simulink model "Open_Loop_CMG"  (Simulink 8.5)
settings: Solver=ode45  StartTime=0.0  StopTime=10000  FixedStep=Ts*5  RelTol=1e-3
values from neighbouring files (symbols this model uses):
  J = [0.119416e9, -0.476e7,   -0.1216e7;     -0.476e7,     0.40408e8, -0.30121e6;     -0.1216e7,   -0.30121e6,  0.110166e9]    [start.m]    (also in start1.m; start2.m; start3.m)
  omg = 20*wo    (= 0.022)    [start.m]    (also in start1.m; start2.m; start3.m)
  wo = 0.0011    [start.m]    (also in start1.m; start2.m; start3.m)
  zeb = 0.95    [start.m]    (also in start1.m; start2.m; start3.m)
undefined symbols (not defined in the file or in its folder): Af, Bf, Cf, Df

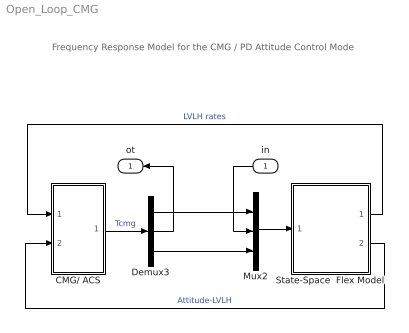
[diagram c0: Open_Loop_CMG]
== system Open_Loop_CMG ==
  note: Frequency Response Model for the CMG / PD Attitude Control Mode
  in : Inport
  CMG/ ACS : Subsystem
  Demux3 : Demux  Outputs=3
  Mux2 : Mux  Inputs=3
  State-Space  Flex Model : Subsystem
  ot : Outport
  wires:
  State-Space  Flex Model/1(w-lv) -> CMG/ ACS/1(wl)  "LVLH rates"
  State-Space  Flex Model/2(att-lv) -> CMG/ ACS/2(ater)  "Attitude-LVLH"
  CMG/ ACS/1(Tq) -> Demux3/1  "Tcmg"
  Mux2/1 -> State-Space  Flex Model/1(Tcmg)
  Demux3/3 -> Mux2/3
  Demux3/1 -> Mux2/1
  Demux3/2 -> ot/1
  in/1 -> Mux2/2

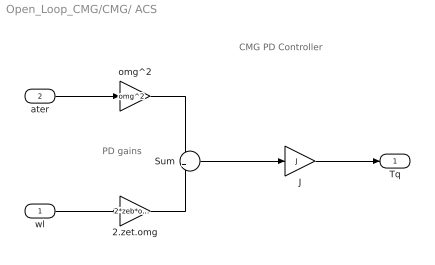
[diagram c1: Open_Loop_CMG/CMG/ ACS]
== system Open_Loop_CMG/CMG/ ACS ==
  note: CMG PD Controller
  note: PD gains
  wl : Inport
  ater : Inport  Port=2  PortDimensions=3
  2.zet.omg : Gain  Gain=2*zeb*omg
  J : Gain  Gain=J  Multiplication=Matrix(K*u)
  Sum : Sum
  omg^2 : Gain  Gain=omg^2
  Tq : Outport
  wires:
  wl/1 -> 2.zet.omg/1
  Sum/1 -> J/1
  2.zet.omg/1 -> Sum/2
  ater/1 -> omg^2/1
  omg^2/1 -> Sum/1
  J/1 -> Tq/1

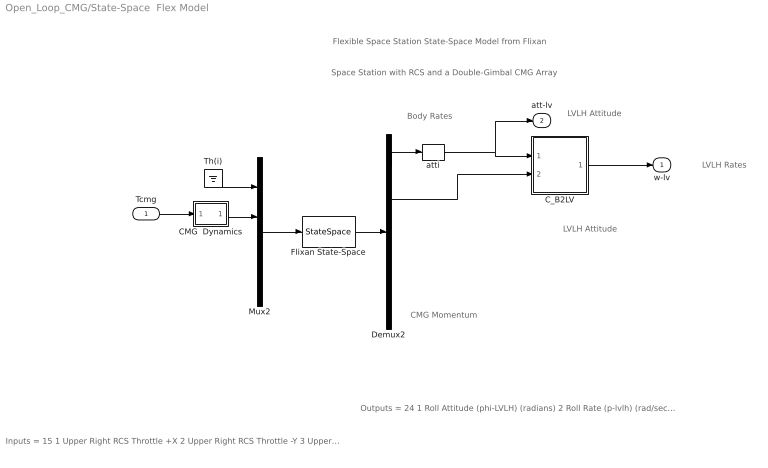
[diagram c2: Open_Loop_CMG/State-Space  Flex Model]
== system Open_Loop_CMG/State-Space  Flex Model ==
  note: Flexible Space Station State-Space Model from Flixan
  note: Space Station with RCS and a Double-Gimbal CMG Array
  note: Body Rates
  note: LVLH Attitude
  note: LVLH Rates
  note: Outputs = 24 1 Roll Attitude (phi-LVLH) (radians) 2 Roll Rate (p-lvlh) (rad/sec) 3 Pitch Attitude (thet-LVLH) (radians) 4 Pitch Rate (q-lvlh) (rad/sec) 5 Yaw Attitude (psi-LVLH) (radians) 6 Yaw Rate (r-lvlh) (rad/sec) 7 Angle of attack, alfa, (radians) 8 Angle of sideslip, beta, (radian) 9 Change in Altitude, delta-h, (feet) 10 Forward Acceleration (V-dot) (ft/sec) 11 Cross Range Velocity (Vcr) (ft/sec) 12 Rate-Gyro # 1, Roll Rate (Body) (rad/sec) 13 Rate-Gyro # 2, Pitch Rate (Body) (rad/sec) 14 Rate-Gyro # 3, Yaw Rate (Body) (rad/sec) 15 Gyro # 4, Roll Attitude (Body) (radians) 16 Gyro # 5, Pitch Attitude (Body) (radians) 17 Gyro # 6, Yaw Attitude (Body) (radians) 18 Accelerom # 1, (along X), (ft/sec^2) Translat. Accelerat. 19 Accelerom # 2, (along Z), (ft/sec^2) Translat. Accelerat. 20 Accelerom # 3, (along X), (ft/sec^2) Translat. Accelerat. 21 Accelerom # 4, (along Z), (ft/sec^2) Translat. Accelerat. 22 Double Gimbal CMG Momentum Change in X-axis (ft-lb-sec) 23 Double Gimbal CMG Momentum Change in Y-axis (ft-lb-sec) 24 Double Gimbal CMG Momentum Change in Z-axis (ft-lb-sec)
  note: LVLH Attitude
  note: Inputs = 15 1 Upper Right RCS Throttle +X 2 Upper Right RCS Throttle -Y 3 Upper Left RCS Throttle +X 4 Upper Left RCS Throttle +Y 5 Lower Right RCS Throttle +X 6 Lower Right RCS Throttle -Y 7 Lower Left RCS Throttle +X 8 Lower Left RCS Throttle +Y 9 Double Gimbal CMG Torque in the X-axis (ft-lb) 10 Double Gimbal CMG Torque in the Y-axis (ft-lb) 11 Double Gimbal CMG Torque in the Z-axis (ft-lb) 12 External Torque Input 1 (ft-lb), direct: 13 External Torque Input 2 (ft-lb), direct: 14 External Torque Input 3 (ft-lb), direct: 15 Ext Torque Direct.=(0.197, -0.5964, -0.7782)
  note: CMG Momentum
  Tcmg : Inport  PortDimensions=3
  CMG  Dynamics : Subsystem
  C_B2LV : Subsystem
  Demux2 : Demux  Outputs=[11, 3, 3, 4, 3]
  Flixan State-Space : StateSpace  A=Af  B=Bf  C=Cf  D=Df  X0=0
  Mux2 : Mux  Inputs=[8, 3, 3, 1]
  Th(i) : Ground
  atti : Selector  InputPortWidth=11  Indices=[1 3 5]
  w-lv : Outport
  att-lv : Outport  Port=2
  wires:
  Mux2/1 -> Flixan State-Space/1
  Flixan State-Space/1 -> Demux2/1
  Tcmg/1 -> CMG  Dynamics/1(I)
  Th(i)/1 -> Mux2/1
  Demux2/1 -> atti/1
  CMG  Dynamics/1(O) -> Mux2/2
  atti/1 -> att-lv/1, C_B2LV/1(atti)
  Demux2/2 -> C_B2LV/2(wb)
  C_B2LV/1(wlv) -> w-lv/1

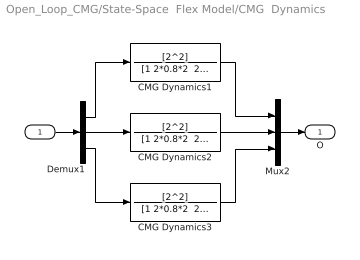
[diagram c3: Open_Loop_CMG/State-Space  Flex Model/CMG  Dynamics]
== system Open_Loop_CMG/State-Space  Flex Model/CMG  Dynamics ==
  I : Inport
  CMG Dynamics1 : TransferFcn  Numerator=[2^2]  Denominator="[1 2*0.8*2  2^2]"
  CMG Dynamics2 : TransferFcn  Numerator=[2^2]  Denominator="[1 2*0.8*2  2^2]"
  CMG Dynamics3 : TransferFcn  Numerator=[2^2]  Denominator="[1 2*0.8*2  2^2]"
  Demux1 : Demux  Outputs=3
  Mux2 : Mux  Inputs=3
  O : Outport
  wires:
  Mux2/1 -> O/1
  I/1 -> Demux1/1
  Demux1/3 -> CMG Dynamics3/1
  Demux1/1 -> CMG Dynamics1/1
  Demux1/2 -> CMG Dynamics2/1
  CMG Dynamics1/1 -> Mux2/1
  CMG Dynamics3/1 -> Mux2/3
  CMG Dynamics2/1 -> Mux2/2

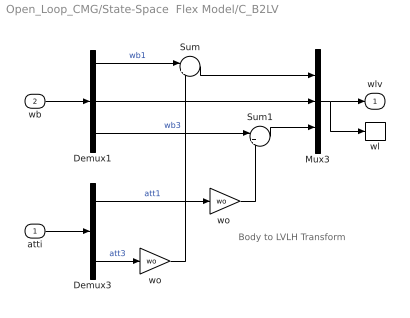
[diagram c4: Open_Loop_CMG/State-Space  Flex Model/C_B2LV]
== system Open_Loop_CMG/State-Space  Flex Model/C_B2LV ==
  note: Body to LVLH Transform
  atti : Inport  PortDimensions=3
  wb : Inport  Port=2  PortDimensions=3
  Demux1 : Demux  Outputs=3
  Demux3 : Demux  Outputs=3
  Mux3 : Mux  Inputs=3
  Sum : Sum  Inputs=|++
  Sum1 : Sum  Inputs=|+-
  wl : ToWorkspace  VariableName=wl  SampleTime=-1
  wo : Gain  Gain=wo
  "wo " : Gain  Gain=wo
  wlv : Outport
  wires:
  Demux1/1 -> Sum/1  "wb1"
  Sum/1 -> Mux3/1
  Demux3/3 -> wo/1  "att3"
  Sum1/1 -> Mux3/3
  atti/1 -> Demux3/1
  wb/1 -> Demux1/1
  Mux3/1 -> wlv/1, wl/1
  Demux3/1 -> "wo "/1  "att1"
  Demux1/2 -> Mux3/2
  wo/1 -> Sum/2
  Demux1/3 -> Sum1/1  "wb3"
  "wo "/1 -> Sum1/2
